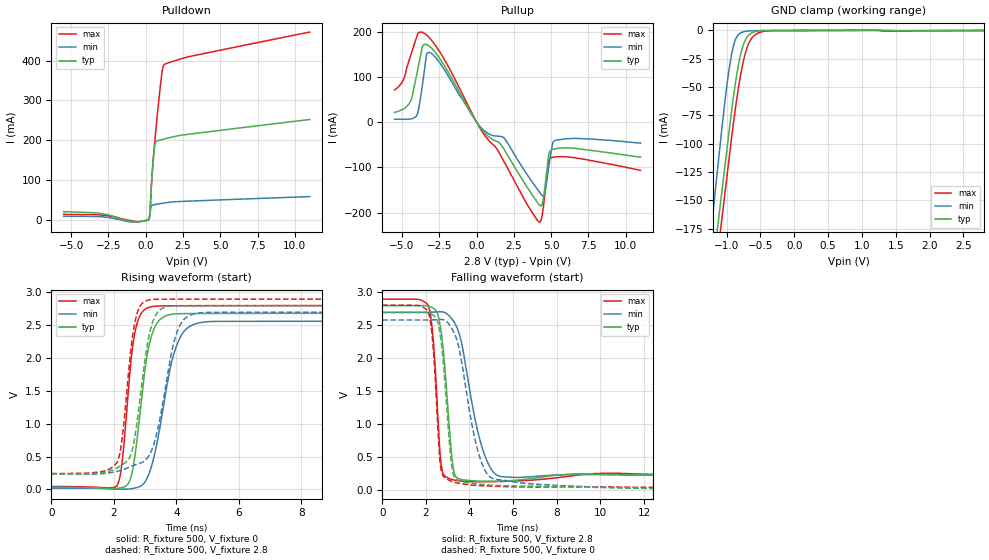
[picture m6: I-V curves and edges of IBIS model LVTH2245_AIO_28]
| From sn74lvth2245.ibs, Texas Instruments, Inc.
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[Model]   LVTH2245_AIO_28
Model_type  I/O
Vinl = 0.8
Vinh = 2.0
Enable   Active-Low
Vref =   0
Rref =   500
Cref =   50p
Vmeas =   1.5
| variable   typ   min   max
C_comp   6.57pF   5.35pF   8.64pF
| C_pullup   5.33pF   0.21pF   8.29pF
| C_pulldown   6.45pF   2.49pF   10.68pF
| C_tri-state   6.57pF   5.35pF   8.64pF
[Temperature Range]   40   -40   100
| Ambient temperature   25   -40   85
[Voltage range]   2.8   2.7   2.9
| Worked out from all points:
|   slope of the pulldown table from 0 to 0.42 V, typ, clamps not added: 3.84 ohm
|   slope of the pullup table from 0 to 0.42 V, typ, clamps not added: 21.7 ohm
|   GND clamp passes 1 mA (typ) near -0.58 V on its own axis
|   rising waveform, R_fixture 500, V_fixture 0: 20-80 % time 421ps typ, 614ps min, 319ps max; typ from 0.031 V to 2.68 V
|   falling waveform, R_fixture 500, V_fixture 2.8: 20-80 % time 381ps typ, 857ps min, 295ps max; typ from 2.8 V to 0.237 V
|   rising waveform, R_fixture 500, V_fixture 2.8: 20-80 % time 449ps typ, 603ps min, 344ps max; typ from 0.238 V to 2.8 V
|   falling waveform, R_fixture 500, V_fixture 0: 20-80 % time 390ps typ, 869ps min, 301ps max; typ from 2.69 V to 0.031 V
[GND Clamp]
| LVTH2245_AIO_28
|   Voltage   I(typ)   I(min)   I(max)
-5.5V     -2.859A    -3.046A    -2.876A
-1.25V    -232.7mA   -189.3mA   -258mA
-1.18V    -197.5mA   -149.1mA   -221.9mA
-1.075V   -144.9mA   -89.41mA   -169mA
-975mV    -95.01mA   -39.15mA   -119.1mA
-925mV    -70.45mA   -20.49mA   -94.22mA
-875mV    -48.53mA   -8.763mA   -71.01mA
-800mV    -22.98mA   -2.372mA   -41.44mA
-725mV    -8.581mA   -848.3uA   -20.47mA
-650mV    -2.878mA   -306.3uA   -8.704mA
-575mV    -968.1uA   -123.1uA   -3.669mA
2.8V      31pA       23.95pA    -464.6pA
[Pulldown]
| LVTH2245_AIO_28
|   Voltage   I(typ)   I(min)   I(max)
-5.5V     21.74mA    10.21mA    15.06mA
-3.065V   17.64mA    9.323mA    13.56mA
-725mV    -3.504mA   -4.492mA   -2.084mA
215mV     2.334mA    2.79mA     2.246mA
285mV     22.68mA    17.65mA    18.48mA
365mV     76.41mA    34.68mA    76.1mA
465mV     132.9mA    38.49mA    134.9mA
620mV     189.7mA    39.6mA     203.1mA
1.05V     201.9mA    42.41mA    358.1mA
1.155V    202.9mA    43.05mA    382.5mA
1.26V     203.9mA    43.67mA    390.4mA
11V       252.5mA    59.6mA     471.2mA
[Pullup]
| LVTH2245_AIO_28
|   Voltage   I(typ)   I(min)   I(max)
-5.5V     21.44mA    6.413mA    70.85mA
-4.465V   43.68mA    6.74mA     142.4mA
-3.99V    108.8mA    16.01mA    191mA
-3.62V    168.2mA    84.82mA    198.4mA
-3.245V   169.8mA    153.9mA    189.4mA
1.895V    -62.93mA   -36.94mA   -90.63mA
4.205V    -183.1mA   -154.4mA   -221.4mA
4.555V    -151.3mA   -159.6mA   -166.9mA
4.815V    -78.5mA    -105.1mA   -88.17mA
5V        -62.26mA   -65.75mA   -79.24mA
5.825V    -56.73mA   -37.54mA   -76.38mA
11V       -77.73mA   -46.53mA   -106.7mA
[Ramp]
| LVTH2245_AIO_28
| variable   typ   min   max
dV/dt_r   1.60/4.24E-10   1.54/6.26E-10   1.67/3.24E-10
dV/dt_f   1.60/3.95E-10   1.51/8.94E-10   1.66/3.05E-10
R_load = 500
[Rising Waveform]
| LVTH2245_AIO_28
R_fixture =   500
C_fixture =   0
L_fixture =   0
V_fixture =   0
V_fixture_min = 0
V_fixture_max = 0
|   Time   V(typ)   V(min)   V(max)
0s        31.45mV    19.46mV    44.09mV
2.1ns     17.17mV    4.869mV    55.22mV
2.26ns    29.34mV    4.277mV    407.1mV
2.46ns    90.88mV    6.686mV    1.488V
2.755ns   821.4mV    32.22mV    2.551V
3.035ns   1.963V     147.2mV    2.756V
3.3ns     2.463V     533.1mV    2.79V
4.025ns   2.675V     2.214V     2.798V
4.93ns    2.681V     2.553V     2.799V
50ns      2.684V     2.563V     2.801V
[Falling Waveform]
| LVTH2245_AIO_28
R_fixture =   500
C_fixture =   0
L_fixture =   0
V_fixture =   2.8
V_fixture_min = 2.7
V_fixture_max = 2.9
|   Time   V(typ)   V(min)   V(max)
0s        2.8V       2.7V       2.9V
2.09ns    2.794V     2.701V     2.811V
2.305ns   2.767V     2.702V     2.403V
2.505ns   2.703V     2.705V     1.401V
2.765ns   2.232V     2.705V     278.9mV
3.175ns   558.3mV    2.607V     168.6mV
3.4ns     199.7mV    2.487V     151mV
4.55ns    140.4mV    681.3mV    131.2mV
5.445ns   142.8mV    210.1mV    135.7mV
50ns      236.9mV    231.2mV    243mV
[Rising Waveform]
| LVTH2245_AIO_28
R_fixture =   500
C_fixture =   0
L_fixture =   0
V_fixture =   2.8
V_fixture_min = 2.7
V_fixture_max = 2.9
|   Time   V(typ)   V(min)   V(max)
0s        237.7mV    231.8mV    243.8mV
2.1ns     327.6mV    275.2mV    409.2mV
2.265ns   377.4mV    298.5mV    780.2mV
2.53ns    516.6mV    349.2mV    2.076V
2.675ns   813.5mV    374.4mV    2.557V
3.175ns   2.445V     563.8mV    2.89V
3.475ns   2.735V     1.084V     2.897V
4.02ns    2.797V     2.398V     2.898V
4.755ns   2.798V     2.69V      2.899V
50ns      2.8V       2.7V       2.9V
[Falling Waveform]
| LVTH2245_AIO_28
R_fixture =   500
C_fixture =   0
L_fixture =   0
V_fixture =   0
V_fixture_min = 0
V_fixture_max = 0
|   Time   V(typ)   V(min)   V(max)
0s        2.695V     2.582V     2.808V
2.085ns   2.689V     2.583V     2.718V
2.295ns   2.663V     2.584V     2.315V
2.5ns     2.591V     2.587V     1.249V
2.715ns   2.217V     2.591V     286.7mV
3.19ns    358.2mV    2.455V     137.2mV
3.63ns    134.6mV    1.969V     102.2mV
4.66ns    89.54mV    337.5mV    69.87mV
6.205ns   66.76mV    119.6mV    54.01mV
50ns      31.44mV    19.41mV    44.11mV
